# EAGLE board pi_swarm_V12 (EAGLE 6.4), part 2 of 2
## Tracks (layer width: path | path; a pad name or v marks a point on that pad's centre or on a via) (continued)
OLED_5  (via drill 0.35 pad 0.7) (continued)
  Bottom 0.2: v66.3,14.5 65.95,14.15 55.35,14.15 54.1,12.9 51.9,12.9 50.65,14.15 49.95,14.15 v49.4,13.6 | v46.05,8.8 42.55,8.8 42.3,9.05 v42.3,10.5
OLED_6  (via drill 0.35 pad 0.7)
  Top 0.2: IO1.9 71.06,31.19 71.4,30.85 v72.1,30.85 | NAND6.12 36.8,6.82 36.8,9.6 37.4,10.2 NAND6.2 37.4,13.76 36.65,14.45 35.8,14.45 35.44,14.09 35.44,13.99 | NAND6.5 35.44,13.99 | 35.44,13.99 35.3,13.85 33.35,13.85 v33.25,13.65
  Bottom 0.2: v72.1,30.85 71.5,30.85 69.75,32.6 29.5,32.6 27.9,31 27.9,15.75 29.75,13.9 33.1,13.9 v33.25,13.65
OLED_7  (via drill 0.35 pad 0.7)
  Top 0.2: IO1.10 71.54,33.11 70.85,33.8 v70.55,33.8 | NAND7.2 v10.65,34.8 10.65,35.3 | NAND7.5 11.01,36.76 10.65,36.4 10.65,35.3 | NAND7.12 10.51,35.44 10.65,35.3
  Bottom 0.2: v70.55,33.8 69.95,33.8 69.3,33.15 29.2,33.15 27.9,31.85 26.8,31.85 25.4,30.45 21.5,30.45 19.85,32.05 18.35,32.05 18.35,35.85 18,36.2 16.8,36.2 16.1,34.95 16.1,32.95 15.65,32.4 13.95,32.4 13.3,33.05 12.4,33.05 v10.65,34.8
OLED_8  (via drill 0.35 pad 0.7)
  Top 0.2: NAND8.2 34.8,89.45 34.65,89.6 33,89.6 32.84,89.44 NAND8.5 32.95,88.42 32.95,87.45 32.9,87.45 32.9,85.35 33.25,85 33.85,85 34.16,84.69 NAND8.12 34.15,80.8 v34.2,80.75 | IO1.12 v72.56,34.3 v72.55,34.3
  Bottom 0.2: v72.55,34.3 72.55,35.4 72.25,35.7 71.55,35.7 71.35,35.9 71.35,35.95 70.15,37.15 70.15,49.4 71.4,50.65 77.4,50.65 78.95,52.2 78.95,72.35 79.3,72.7 79.3,75 77.75,76.55 76.85,76.55 75,78.4 75,80.4 74.85,80.55 38.5,80.6 37.8,81.3 34.75,81.3 v34.2,80.75
OLED_9  (via drill 0.35 pad 0.7)
  Top 0.2: IO1.13 73.04,33.49 73.5,33.95 74.35,33.95 v75.2,34.8 | NAND9.12 43.49,83.59 v44,84.1 | NAND9.5 42.17,89.77 42.4,90 v43.95,90 44.13,89.82 NAND9.2
  Bottom 0.2: v43.95,90 44.7,89.25 44.7,85.25 44,84.55 v44,84.1 44.3,84.1 44.55,84.35 45.75,84.35 46.1,84 46.1,83.4 45.3,82.6 45.3,81.4 45.7,81 75.1,81 75.45,80.65 75.45,78.65 77.1,77 78,77 79.75,75.25 79.75,72.5 79.4,72.15 79.4,51.95 77.6,50.15 71.65,50.15 70.6,49.1 70.6,37.35 71.8,36.15 74.4,36.15 75.2,35.35 v75.2,34.8
OLED_10  (via drill 0.35 pad 0.7)
  Top 0.2: IO1.14 73.55,33.3 73.75,33.5 75,33.5 75.6,34.1 76.3,34.1 v76.5,34.25 | 52.85,84.3 v53.5,84.3 52.83,84.28 NAND10.12 | NAND10.2 53.46,89.69 53.15,90 v53.15,90.3 52.25,90.3 51.51,89.56 NAND10.5
  Bottom 0.2: v76.5,34.25 76.5,35.45 75.35,36.6 72.05,36.6 71.05,37.6 71.05,48.85 71.9,49.7 77.95,49.7 79.85,51.65 79.85,72 80.2,72.35 80.2,75.55 78.3,77.45 77.35,77.45 75.9,78.9 75.9,80.9 75.35,81.45 57.4,81.45 56.15,82.7 56.15,83.6 55.95,83.8 53.95,83.8 v53.5,84.3 53.5,85.1 53.95,85.55 53.95,86.95 53.85,87.05 53.85,90.05 53.6,90.3 v53.15,90.3
OLED_B  (via drill 0.35 pad 0.7)
  Top 0.2: NAND1.4 61.5,85.65 61.1,85.25 59,85.25 58.2,84.5 56.5,84.5 55.35,85.65 52.7,85.65 52.17,86.18 NAND10.4 52.17,86.52 52.1,86.45 50.65,86.45 50.6,86.4 42.88,86.4 42.83,86.45 | NAND8.4 33.5,85.6 33.65,85.45 36.1,85.45 36.1,82.3 36.4,82 36.5,82 | v35.8,10.8 36.1,11.1 NAND6.4 v36.1,13.8 | v46.1,10.9 NAND5.4 | 36.5,82 37.1,82 37.4,82.3 37.4,88.2 37.8,88.6 39.4,88.6 39.95,88.05 39.95,86 40.15,85.8 42.18,85.8 42.83,86.45 | v16.7,44.1 16.7,43.4 16.85,43.25 16.85,36.1 16.45,35.7 16.45,35.65 | v84.85,58.85 84.85,59.15 84.75,59.25 NAND2.4 | NAND4.4 56.1,11.6 v55.65,11.15 | v31.95,63.75 31.85,63.85 31.85,71 32.9,72.05 32.9,76.15 33.1,76.35 v33.1,79.3 | v36.1,80.35 36.1,81.55 36.5,82 | NAND3.4 81.3,27.45 v81.45,27.3 | v68.05,12.15 v66.3,12.15 | v16.65,32.15 21.05,32.15 21.35,32.45 21.35,33.25 26,33.25 26.4,33.65 26.4,34.2 26.7,34.5 27.7,34.5 28,34.2 28,30.65 v28.55,30.1 | NAND9.4 42.83,86.45 | NAND7.4 15.3,36.1 16.1,35.65 16.45,35.65 | 16.45,35.65 16.45,35.4 v16.85,34.9
  Bottom 0.2: v35.8,10.8 36.2,11.2 45.8,11.2 v46.1,10.9 46.35,11.15 v55.65,11.15 56.3,10.45 58,10.45 58.2,10.3 60.4,10.3 60.8,10.05 65.75,10.05 66.3,10.6 v66.3,12.15 | v16.7,44.1 21.05,44.1 21.55,44.5 23,45.65 23,48.6 24.05,49.65 28.5,49.65 31.85,53 MBED.P24 31.85,63.65 v31.95,63.75 | v84.85,58.85 84.85,58.7 84.4,58.25 81.95,58.25 81.4,57.7 81.4,50.75 78.4,47.75 78.4,40.2 81.45,37.5 81.8,37.15 81.8,27.65 v81.45,27.3 81.5,27.3 81.6,27.4 87.65,27.4 88.15,26.9 88.15,26.35 87.7,25.9 84.1,25.9 74.65,16.45 69.35,16.45 68.05,15.15 v68.05,12.15 67.75,12.15 | v33.1,79.3 33.6,79.8 35.55,79.8 v36.1,80.35 | v16.85,34.9 16.85,34.5 16.7,34.35 16.7,32.2 v16.65,32.15 | v28.55,30.1 28.55,16.45 30.6,14.4 35.55,14.4 v36.1,13.8
OLED_G  (via drill 0.35 pad 0.7)
  Top 0.2: NAND1.13 62.8,81.59 | 62.8,81.59 62.2,81 58.55,81 58.05,81.5 58.05,83.25 57.85,83.45 56.95,83.45 54.5,81 53.51,81 53.46,81.05 | 44.15,81 38,81 | NAND8.13 34.8,81.4 35.4,80.8 35.4,80.1 35.85,79.65 37.2,79.65 37.7,80.15 37.7,80.8 37.9,81 38,81 | NAND9.13 44.13,81.02 44.15,81 | NAND10.13 53.46,81.05 | 53.46,81.05 53.46,81.01 53.45,81 49.8,81 49.6,81.2 49.6,82.9 49.3,83.5 46.9,83.5 45.4,82.1 45.4,81 44.15,81 | NAND5.13 47.4,9.1 v47.65,9.35 47.5,9.5 45.55,9.5 45.45,9.4 v45.45,8.15 | v57.4,9.35 NAND4.13 | v23.2,41.35 22.8,41.35 21.6,42.55 18.5,42.55 18.15,42.2 v18.15,41.85 | NAND7.13 9.45,34.8 11.3,32.95 11.3,31.85 11.7,31.45 | v32.75,62.4 v32.75,65.9 | v38.1,72.25 38.1,80.9 38,81 | NAND6.13 37.4,7.89 v37.65,8.15 | v14.75,33.45 12.65,31.35 11.8,31.35 11.7,31.45 | v28.3,7.9 v28.3,9.7 | v5.25,29.7 9.95,29.7 11.7,31.45 | 62.8,81.59 62.8,80.45 63.85,79.4 63.85,71.4 v64.85,70.4 | v77.7,66.95 80,66.95 80.65,66.3 81.8,66.3 v81.9,66.4 | v90.85,55.2 90.45,55.2 88.45,53.2 84.4,53.2 84.25,53.05 83.25,53.05 v83.1,52.9 | v84.45,28.75 NAND3.13 | v87.85,60.55 NAND2.13 v87.86,60.55 v87.85,60.55
  Bottom 0.2: v47.65,9.35 v57.4,9.35 | v18.15,41.85 16.35,41.85 15.5,41.5 15.5,40.5 16.35,39.8 16.35,36.35 15.55,34.9 15.4,34.75 14.75,34.75 v14.75,33.45 | v23.2,41.35 25.05,43.25 29.85,43.25 29.85,50.2 31.85,52.2 33.8,52.2 34.39,52.79 MBED.P25 34.34,61.11 v32.75,62.4 | v32.75,65.9 32.75,70.35 34.5,72.1 37.95,72.1 v38.1,72.25 | 38.9,8.15 v45.45,8.15 | v37.65,8.15 38.9,8.15 | 38.9,8.15 38.9,5.8 38.6,5.5 33.25,5.5 32.8,5.95 32.8,7.65 32.55,7.9 v28.3,7.9 | v28.3,9.7 23.1,9.7 22.65,9.25 21.8,9.25 19.85,10.5 17.5,12.3 14.85,14.85 14.8,15.85 11.95,18.65 12,21.5 5.75,27.7 5.75,29.2 v5.25,29.7 | v64.85,70.4 74.25,70.4 v77.7,66.95 | v81.9,66.4 82.5,65.8 83.65,65.8 85.65,67.4 85.65,68.95 85.95,69.25 87.7,69.2 88.15,67.6 88.15,60.85 v87.85,60.55 87.85,56.9 88.2,56.55 89.8,55.2 v90.85,55.2 | v83.1,52.9 82.4,52.2 82.4,50.05 79.5,47.1 79.5,40.85 82.55,38.15 82.65,38.05 82.95,38.05 83.25,37.75 83.25,35.65 83.4,35.5 83.4,29.8 v84.45,28.75
OLED_R  (via drill 0.35 pad 0.7)
  Top 0.2: v41.95,90.65 44.6,90.65 45.35,89.9 45.35,88.5 45.27,88.42 NAND9.1 44.79,87.56 v45.3,87.05 | v36.7,88.4 35.48,88.4 NAND8.1 | NAND10.1 55.02,88.42 v55.2,88.6 | NAND1.1 63.46,86.89 v63.8,86.55 | 38.05,14.15 NAND6.1 | NAND5.1 48.06,13.89 48.02,13.93 | 48.02,13.93 47.65,14.25 38.15,14.25 38.05,14.15 | NAND4.1 58.06,13.84 | 58.06,13.84 57.65,14.25 48.35,14.25 48.02,13.93 | NAND7.1 13.73,34.2 17.6,34.2 18.25,34.85 18.25,36.05 18.05,36.25 18.05,41.15 18.35,41.15 18.65,41.4 18.85,41.7 18.85,42.15 21.35,42.15 22.9,40.6 27.35,40.6 27.45,40.5 | MBED.P26 36.93,56.07 36.9,56.1 | 38.05,14.15 37.65,14.15 36.9,14.9 35.6,14.9 35,14.3 31.3,14.3 30.25,15.35 30.25,37.7 28.5,39.45 27.8,39.45 27.45,39.8 27.45,40.5 | 58.06,13.84 62.84,13.84 63.8,14.8 63.8,15.1 v64.45,15.7 | v66.75,19.3 66.75,20.7 66.95,20.9 67.5,20.9 68.05,21.45 v70.25,21.45 | v79.35,23.75 79.7,23.75 v80.65,24.7 | v81.15,29.4 NAND3.1 | 36.9,56.1 36.2,56.8 23.95,56.8 22.7,55.55 22.7,43 23,42.7 25.4,42.7 25.5,42.8 26.25,42.8 26.3,42.75 27.2,42.75 27.45,42.5 27.45,40.5 | 36.9,56.1 v37.3,56.5 43.15,56.5 43.8,55.85 v48.45,55.85 | v37,64.2 37,69.1 v38.35,70.45 | v40.75,74.9 40.75,79.85 41,80.1 43,80.1 43.3,79.8 43.3,73.85 43.65,73.5 45.6,73.5 45.9,73.8 45.9,79.6 46.5,80.2 v46.5,81.6 | NAND2.1 81.06,61.21 77.9,58.05 75.6,58.05 75.45,57.9 75.45,55.45 v75.3,55.3
  Bottom 0.2: v36.7,88.4 37,88.7 37,90.1 37.55,90.65 v41.95,90.65 42.65,91.35 44.7,91.35 45.15,91.8 45.15,92.3 45.55,92.7 46.5,92.7 46.85,92.35 52.7,92.35 53.2,91.85 53.2,91.2 53.35,91.05 54.25,91.05 55.2,90.1 v55.2,88.6 55.25,88.55 55.25,85.35 55.75,84.85 57.25,84.85 57.65,85.25 57.65,86.8 58.15,87.3 63.05,87.3 v63.8,86.55 | v64.45,15.7 64.7,15.9 65.1,16.2 65.1,17.65 v66.75,19.3 | v70.25,21.45 70.25,26.8 71.4,27.95 75.95,27.95 76.5,28.5 77.6,28.5 77.95,28.15 77.95,25.05 79.25,23.75 v79.35,23.75 | v80.65,24.7 80.65,28.9 v81.15,29.4 | v37.3,56.5 37.3,63.9 v37,64.2 | v38.35,70.45 40.75,72.85 v40.75,74.9 | v45.3,87.05 45.3,85.8 46.5,84.6 v46.5,81.6 | v75.3,55.3 75.05,55.3 74.65,55.7 48.6,55.7 v48.45,55.85
SCL  (via drill 0.35 pad 0.7)
  Top 0.2: IO1.2 67.55,33.6 66.8,34.35 66.6,34.35 v65.9,35.05 | R15.1 59.1,47.45 v59.1,44.75 59.15,44.8 61.45,44.8 62.95,46.3 v62.95,49.45 62.95,49.75 62.95,50 61.25,51.7 60.8,51.7 | MBED.P27 39.47,55.52 39.65,55.7 43,55.7 43.25,55.45 43.25,51.85 43.4,51.7 60.8,51.7 | v58.45,62.95 58.64,63.14 ADC1.19 61.51,63.14 v61.55,63.1 | v60.75,68 60.75,68.8 60.95,69 MAGNETO.7 | v61.45,57.35 61.1,57 v61.1,55 | v60.8,51.2 60.8,51.7 | EEPROM.1 77.52,53.17 v78.1,53.75 | v70.1,51.1 68.5,51.1 v66.9,49.5
  Bottom 0.2: v65.9,35.05 65.9,42.05 63.2,44.75 61.95,44.75 | 61.95,44.75 v59.1,44.75 | v58.45,62.95 58.45,65.7 v60.75,68 | v61.55,63.1 61.55,57.45 v61.45,57.35 | v61.1,55 61.1,51.5 v60.8,51.2 | I2C_CONN.P$3 62.1,44.6 61.95,44.75 | v78.1,53.75 75.9,51.55 70.55,51.55 v70.1,51.1 | v66.9,49.5 63,49.5 v62.95,49.45
SDA  (via drill 0.35 pad 0.7)
  Top 0.2: IO1.1 65.66,32.24 64.2,33.7 v64.2,35.05 | v57.5,44.75 57.5,49.05 57.83,49.38 | 57.83,49.38 58.35,49.9 R14.1 | MBED.P28 42.01,51.69 42.45,51.25 55.95,51.25 57.12,50.08 | 57.12,50.08 57.83,49.38 | ADC1.18 58.98,62.48 v58.45,61.95 | v63.2,68.6 MAGNETO.6 | v59.1,57.1 59.1,57.05 58.5,56.45 v58.5,52.9 | v57.75,50.8 57.75,50.7 57.12,50.08 | EEPROM.3 74.66,53.79 74.05,54.4 74.05,57.3 v73.15,58.2
  Bottom 0.2: v64.2,35.05 64.2,38.05 63.8,38.05 62.3,39.55 60.6,39.55 60.1,40.05 I2C_CONN.P$2 60.1,42.15 v57.5,44.75 | v63.2,68.6 63.2,66.65 58.5,61.95 v58.45,61.95 58.45,60.4 59.1,59.75 v59.1,57.1 59.55,56.65 72.2,56.65 73.15,57.6 v73.15,58.2 | v58.5,52.9 58.5,51.55 v57.75,50.8
TEMP
  Top 0.2: MBED.P20 24.23,76.58 23.6,75.95 21.45,75.95 20.4,77 18.85,77 18.5,77.35 TEMP.3
TRIG
  Bottom 0.2: SONAR_CON.TRIG 46.23,56.87 47.1,56 MBED.P30
USBD+
  Top 0.2: R64.1 40.3,34.65 39.8,34.15 38.4,34.15 37.75,34.8 37.75,40.8 34.45,44.1 USB_CONNECTOR.PIN3
  Bottom 0.2: USB_CONNECTOR.PIN3 37.15,44.1 37.9,43.35 37.9,40.6 39.35,39.15 48.1,39.15 48.75,39.8 48.75,53.64 MBED.P31
USBD-  (via drill 0.35 pad 0.7)
  Top 0.2: v38.95,35 R63.1
  Bottom 0.2: USB_CONNECTOR.PIN2 37.2,42.1 37.4,41.9 37.4,40.4 39.15,38.65 | MBED.P32 51.3,53.65 51.3,39.3 50.65,38.65 39.15,38.65 | 39.15,38.65 39.15,35.2 v38.95,35
V3.3  (via drill 0.35 pad 0.7)
  Top 0.2: C1.1 25.72,74.13 26.65,73.2 ACCEL.2 29.55,73.2 ACCEL.15 ACCEL.16 | C1.1 C2.1 26.48,71.47 v26.7,71.25 | TEMP.4 22.54,77.99 22.95,78.4 22.95,79.25 23.55,79.85 25.1,79.85 25.5,79.45 | 25.5,79.45 25.5,76.25 25.15,75.9 C1.1 | GYRO.9 49.7,67.1 49.9,67.3 49.9,68.95 49.55,69.3 GYRO.1 48.85,70.5 | MAGNETO.2 60.5,69.8 60.9,69.4 MAGNETO.8 63.9,69.4 64.15,69.15 64.15,66.7 63.95,66.5 | IO1.18 75.55,33.25 75.8,33.5 77.6,33.5 77.8,33.7 v77.8,34.25 | v72.05,38.4 IO1.46 | R15.2 R14.2 60.75,48.75 60.8,48.7 v62,48.7 | MBED.P40 72.5,56.3 71.4,57.4 R29.1 66.85,58.3 66.5,58.65 64.3,58.65 63.9,59.05 63.9,63.3 | 72.5,54 MBED.P40 | MBED.P40 | R32.1 6.85,51.75 9.15,54.05 v9.95,54.05 | v9.95,44.35 9.95,47.26 ALPHA433.9-VDD | ADC1.2 57.16,63.14 57.2,63.1 | 57.2,63.1 57.2,62.15 | 57.2,62.15 57.2,61.2 57.1,61.1 54.56,61.1 | 54.56,61.1 ADC1.5 | 54.56,61.1 54.56,60.6 ADC1.6 | C4.1 63.9,63.3 | 63.9,63.3 64.2,63.6 64.2,66.25 63.95,66.5 | 63.95,66.5 C3.1 62.8,66.45 57.7,66.45 57.2,65.95 57.2,63.1 | v44.55,93.1 44.2,92.75 R23.1 44.15,92.75 46.25,90.55 46.25,88.75 v47.7,87.45 | v57,86 57,87 R17.1 | R38.1 v59.9,9.15 59.9,2.95 59.3,2.35 59.05,2.25 50.85,2.25 v50.85,1.6 | v66.75,17.1 v68.1,17.1 | v77.1,27.85 77.1,28.35 v79.35,30.45 | v80.5,35.85 82.7,35.85 | 82.7,35.85 90.75,35.85 92.35,37.45 92.35,38.2 92.7,38.55 92.7,40.9 R26.1 | 48.85,70.5 47.6,71.75 39.15,71.75 38.5,71.1 37.7,71.1 37.4,70.8 36.35,70.8 35.7,71.45 35.7,79.05 34.8,79.95 32.65,79.95 32.55,79.85 25.9,79.85 25.5,79.45 | v27.35,67.65 25.8,67.65 R20.1 25.5,67.85 v25.5,69 | v76.3,55.2 76.75,54.75 81.7,54.75 v82.25,54.2 | v82.55,37.4 82.55,36 82.7,35.85
  Top 0.2: v31.85,6.65 31.85,7.4 29.7,9.55 29.7,13.75 29.05,14.4 26.75,14.4 26.25,13.9 R35.1 | 48.85,70.5 49.35,71 v49.4,71 | v56.3,62.1 57.15,62.1 57.2,62.15 | v48.45,82.35 48.45,80.6 48.6,80.45 v48.6,73.45 | IO1.56 67.04,43.91 v66.7,44.25 59.8,44.25 58.1,42.55 I2C_CONN.P$1 | LIGHTSENSOR.P$1 25,51.25 24.75,51.25 24.25,51.75 v23.65,51.75 | v19.35,51.8 v19.35,54.05 | R42.2 64.6,47.6 64.55,47.6 v64.1,48.05 | EEPROM.4 68.88,50.43 v68.33,49.88
  Bottom 0.2: v72.05,38.4 73.4,37.05 75.75,37.05 77.8,35 v77.8,34.25 79.35,34.25 | v62,48.7 64.2,48.7 | 64.2,48.7 67.15,48.7 v68.33,49.88 68.38,49.92 68.38,52.33 68.45,52.4 71.75,52.4 72.5,53.15 72.5,54.45 | 72.5,54.45 MBED.P40 | v9.95,44.35 v9.95,54.05 19.25,54.05 | v44.55,93.1 44.65,93.2 52.75,93.2 53.9,92.05 53.9,91.7 54.05,91.55 54.55,91.55 55.95,90.15 55.95,86.2 56.15,86 v57,86 | v59.9,9.15 67.25,9.15 67.25,9.9 66.95,10.2 66.95,16.8 66.7,17.05 v66.75,17.1 | v68.1,17.1 74.5,17.1 76.6,19.2 76.6,27.35 v77.1,27.85 | v79.35,30.45 79.35,34.25 | 79.35,34.25 79.35,34.8 v80.5,35.85 | 19.25,54.05 v19.35,54.05 | v19.35,54.05 19.7,54.05 27.15,61.5 27.15,67.45 v27.35,67.65 | v26.7,71.25 26.7,70.1 25.6,69 v25.5,69 | 72.5,54.45 72.65,54.6 75.7,54.6 v76.3,55.2 | v82.25,54.2 81.9,53.85 81.9,50.4 78.95,47.45 78.95,40.6 81.95,37.95 v82.55,37.4 | v50.85,1.6 45.2,1.6 44.2,2.6 38.8,2.6 38.6,2.4 36.45,2.4 35.55,3.3 32.6,3.3 31.85,4.05 v31.85,6.65 | v56.3,62.1 55.35,61.15 48.8,61.15 48.55,61.4 48.55,66.35 49.4,67.2 v49.4,71 48.6,71.8 v48.6,73.45 | v47.7,87.45 47.7,85.9 48.5,85.1 v48.45,82.35 48.5,82.25 | v66.7,44.25 66.7,46.25 64.73,48.18 | 64.73,48.18 64.2,48.7 | v23.65,51.75 19.4,51.75 v19.35,51.8 | 19.25,54.05 19.35,54.15 v19.35,54.05 | v64.1,48.05 64.49,48.4 64.73,48.18
V_IR  (via drill 0.35 pad 0.7)
  Top 0.2: REG1.5 72.71,69.79 C13.1 72.65,71.65 v72.25,72.05 | R24.1 30.05,89.1 v30.8,88.35 | v38.1,87.95 v38.1,82.6 38.1,82.25 37,81.15 v37,80.35 | v67.85,72.05 R18.1 | R30.1 v87.9,70 | v82.3,69.15 v77.8,69.15 | R27.1 90.65,54.05 v90.3,53.7 | v64.95,72.05 v64.95,74.4 | v53.4,79.3 53.4,79.35 53.85,79.8 54.3,79.8 v56.2,81.65 | v47.65,84.9 47.45,85.1 45.45,85.1 v45.45,83.65 | R36.1 36.1,4 36.3,3.8 v36.75,3.8 | v44.9,3.95 44.9,3.15 v45.55,2.5 | v58.9,3 58.9,9.6 60.15,10.85 60.85,10.85 v60.95,10.75 | v63.45,13.05 63.45,13.8 v64.45,14.8 | v66.75,18.1 68.4,18.1 68.9,17.6 68.9,15.4 v69.35,15 | R39.1 70.6,11.8 70.7,11.85 71.25,12.4 v71.25,15 73.5,15 v75.6,12.85 | v91.95,51.05 91.8,50.9 91.8,43.5 91.65,43.35 91.65,37.5 90.95,36.8 v90.3,36.8 | R33.1 2.25,39.85 2.6,39.5 9,39.5 10.95,41.45 10.95,43.3 v11.2,43.55 | R21.1 25.75,61.9 26.25,61.45 v28.5,61.45 33.5,61.45 33.8,61.75 33.8,71.35 33.55,71.6 33.55,73.85 33.8,74.1 v33.8,75.9
  Bottom 0.2: v30.8,88.35 35.05,88.35 35.7,87.7 37.85,87.7 v38.1,87.95 | v82.3,69.15 82.45,69.2 83.6,69.2 84.4,70 v87.9,70 88.25,70 88.65,69.6 88.65,66 90.65,64.4 91.95,60.55 91.95,55.35 v90.3,53.7 90.3,52.7 v91.95,51.05 | v77.8,69.15 77.3,69.15 74.25,72.2 72.4,72.2 v72.25,72.05 v67.85,72.05 v64.95,72.05 | v64.95,74.4 58.1,74.4 56.85,75.65 54.9,75.65 53.4,77.15 v53.4,79.3 | v56.2,81.65 56.05,81.5 48.2,81.5 47.8,82.1 47.8,84.75 v47.65,84.9 | v45.45,83.65 44.4,82.6 v38.1,82.6 | v36.75,3.8 36.9,3.95 v44.9,3.95 | v45.55,2.5 58.4,2.5 v58.9,3 | v60.95,10.75 60.95,11.05 63.15,11.05 63.45,11.35 v63.45,13.05 | v64.45,14.8 66.1,16.45 66.1,17.5 v66.75,18.1 | v69.35,15 v71.25,15 | v90.3,36.8 90.3,29.65 89.45,27.75 88.35,25.65 85.25,20.9 82.35,17.3 79.2,14.2 77.55,12.65 75.8,12.65 v75.6,12.85 | v11.2,43.55 11.2,44.75 27.3,60.85 27.85,60.85 v28.5,61.45 | v37,80.35 37,80.15 35.7,78.85 35.7,75.9 35.6,75.8 33.9,75.8 v33.8,75.9
V_LED  (via drill 0.35 pad 0.7)
  Top 0.2: REG2.5 C14.1 66.6,71.8 66.15,72.25 66.15,81.95 65.52,82.58 NAND1.14 63.46,82.6 v64.5,82.6 | v86.55,61.2 86.69,61.21 NAND2.14 89.9,61.2 v90.2,60.05 LED2.PIN2 | NAND10.14 55.13,82.58 56.12,83.58 | v58.75,82.6 58.75,83.3 58.1,83.95 56.5,83.95 56.12,83.58 | v38.1,3.25 38.1,2.9 39.5,1.5 LED5.PIN2 | v38.1,3.25 38.1,6.74 NAND6.14 | NAND5.14 48.06,5.46 v47.8,5.2 | NAND3.14 86.9,29.4 87.45,29.75 v87.45,30.3 88.7,30.3 | v6.15,34.15 NAND7.14 | NAND4.14 v58.06,5.36 v58.05,5.35 58.15,5.45 | v14.5,19.45 12.97,17.92 13,16.5 13.25,16.05 15.45,13.7 17.9,11.5 18.23,11.17 LED6.PIN2 | v39.45,12.3 39.45,4.6 v38.1,3.25 | v84.05,53.85 88.45,53.85 90.2,55.65 v90.2,58.3 | v68.05,11 67.85,11 67.35,11.5 63.35,11.5 63.35,6.2 63.3,6.2 v63.05,5.95 | NAND8.14 35.46,84.14 v35.25,84.35 | v41.8,84.6 42.3,84.6 42.5,84.8 44.3,84.8 44.75,84.35 44.75,82.62 NAND9.14 45.28,82.58 46.1,83.4 46.1,84.2 46.25,84.35 47.25,84.35 47.45,84.15 48,84.15 49.05,85.2 53.85,85.2 v54.5,84.55 55.48,83.58 56.12,83.58 | v21.45,81.85 20.65,80.9 17.4,80.9 16.2,79.7 16.2,78.2 v15.45,77.45 | v77.05,80.1 77.55,80.1 78.48,81.03 78.1,82.15 LED1.PIN2 | v54.55,89.8 54.55,91.65 54.2,92 52.7,92 52.6,92.1 50.4,92.1 LED10.PIN2 | 88.7,30.3 89.23,30.3 LED3.PIN2 | 88.7,30.3 88.9,30.1 88.9,28.37 88.15,26.85 88.15,24.2 87,22.3 85.6,20.3 84.1,18.4 82.45,16.45 79.2,13.05 77.85,11.8 76.7,10.8 73.85,8.7 LED4.PIN2 v71.8,8.15 | LED7.PIN2 3.29,34.96 2.75,35.5 2.75,38.4 3.05,38.7 v4.35,38.7 | v17.3,70.75 17.3,69.35 14.15,65.95 11.1,65.95 v10.8,66.2 | v5.35,63.75 4.8,63.73 LED8.PIN2 | LED9.PIN2 v22.05,86.7
  Bottom 0.2: v58.75,82.6 v64.5,82.6 65.15,81.95 75.65,81.95 76.45,81.15 76.45,80.15 | v86.55,61.2 86.15,61.2 84.1,63.2 82.25,63.2 81.65,63.75 81.65,65.55 81.2,66 80.55,66 80.3,66.25 80.3,71.75 80.7,72.15 80.7,75.7 78.5,77.9 77.65,77.9 76.45,79.1 76.45,80.15 | v38.1,3.25 38.2,3.15 47.2,3.15 47.8,3.75 v47.8,5.2 47.95,5.35 54.7,5.35 | v4.35,38.7 4.35,34.55 4.75,34.15 v6.15,34.15 5.9,33.9 5.9,31.2 6.3,30.8 6.3,27.95 14.5,19.75 v14.5,19.45 24.35,19.5 25.1,18.8 25.05,14.6 26.75,12.8 39,12.75 v39.45,12.3 | v58.05,5.35 54.7,5.35 | v87.45,30.3 87.45,35.55 86.55,36.45 84.15,36.45 83.95,36.65 83.95,37.8 83.2,38.55 83,38.55 80.05,41.1 80.05,46.95 82.9,49.85 82.9,51.9 83.2,52.2 83.6,52.2 83.85,52.45 83.85,53.2 83.95,53.3 v84.05,53.85 | v68.05,11 71.4,8.9 71.4,8.45 v71.8,8.15 | v63.05,5.95 63.05,4.7 62.05,3.7 54.7,3.7 54.7,5.35 | v41.8,84.6 35.85,84.6 35.6,84.35 v35.25,84.35 34.95,84.35 34.6,84 27.4,84.05 27.05,84.4 26.6,84.4 26,84.65 25.35,84.65 | v21.45,81.85 24.25,84.65 25.35,84.65 | v77.05,80.1 76.5,80.1 76.45,80.15 | v54.55,89.8 54.5,89.75 v54.5,84.55 | v90.2,60.05 v90.2,58.3 | v15.45,77.45 14.25,76.25 14.25,72.6 14.65,72.2 15.05,72.2 16.8,70.75 v17.3,70.75 | v10.8,66.2 10.55,66.2 9.9,65.55 7.15,65.55 v5.35,63.75 | v22.05,86.7 25,86.7 25.5,86.2 25.5,84.8 25.35,84.65
VBAT  (via drill 0.35 pad 0.7)
  Top 0.2: REG2.1 66.65,64.34 66.65,63.45 65.35,62.15 65.35,60.4 C9.1 65.3,59.3 65.45,59.15 | REG1.1 72.7,62.2 72.35,61.85 C11.1 72.35,59.4 72.05,59.1 65.5,59.1 65.45,59.15 | 65.45,59.15 68.9,59.15 68.9,58.35 71.7,58.35 73.5,56.55 73.5,52.65 72.8,51.95 67.8,51.95 v66,50.15 | v55.55,39.6 45.75,39.6 v44.95,40.4
  Bottom 0.2: v66,50.15 58.65,50.15 56.75,48.25 56.75,40.8 v55.55,39.6 | v44.95,40.4 3PI_HEADER.P$12
VBOOST  (via drill 0.35 pad 0.7)
  Top 0.2: v43.25,62.3 44,62.3 45.05,63.35 v49.55,63.35
  Bottom 0.2: 3PI_HEADER.P$13 42.42,45.97 42.85,46.4 43.4,46.4 43.7,46.7 43.7,52.3 43.25,52.75 v43.25,62.3 | v49.55,63.35 50.9,63.35 52,64.35 52,68 53.2,69.2 56.95,69.2 60.65,72.95 68.7,72.95 70,74.25 70,77.33 MBED.P2
VCC
  Bottom 0.2: USB_CONNECTOR.PIN1 31.5,39.6 30.6,40.5 30.6,50.1 31.95,51.45 33.95,51.45 34.35,51.85 40.75,51.85 41.15,51.45 41.15,40 41.5,39.65 47.25,39.65 47.5,39.9 3PI_HEADER.P$11 47.55,43.1 47.55,45.9 47.45,46 46.45,46 46.2,46.25 46.2,52.3 46.1,52.4 46.1,55.4 45.45,56.05 45,56.05 44.75,56.3 44.75,57.55 44.65,57.65 44.1,57.65 44,57.75 44,70.1 44.5,70.6 44.5,72.75 43.7,73.55 SONAR_CON.VCC

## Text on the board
Top: TOP | JAH-2013
Bottom: BOTTOM | pi-swarm | YRL
tNames: LED10 | LED1 | LED9 | LPC1768 MBED | - | GYRO | CHG | + | MAG | LED2 | + | LED8 | JAH-2013 | ALPHA TRX-433 | RF TX | LIGHT / SENSOR | CENTRE | LED | York Robotics / Laboratory | V+ | SDA | SCL | GND | C:/Users/jah128/Desktop/University of York logo black.bmp | ANT | I²C OUT | USB | ID / SWITCHES | LED7 | 16 | 8 | 4 | 2 | 1 | LED3 | PCB Version 1.2 | POWER | Pi Swarm Board | LED6 | LED4 | LED5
